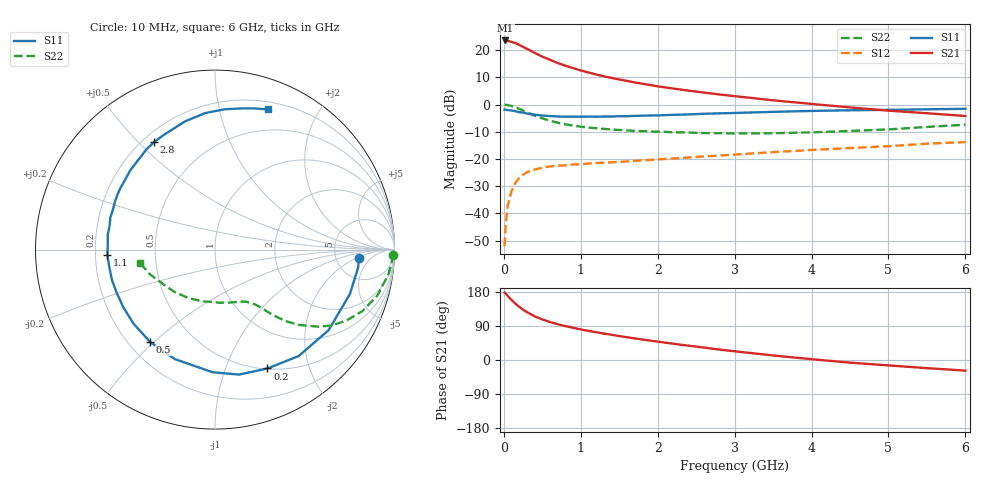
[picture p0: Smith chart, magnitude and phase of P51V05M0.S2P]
! SIEMENS Small Signal Semiconductors
! BFP183
! Si NPN RF Bipolar Junction Transistor in SOT143
! VCE = 1 V  IC = 5 mA
! Common Emitter S-Parameters:  March  1996
# GHz  S  MA  R  50
!  f  S11  S21  S12  S22
! GHz  MAG  ANG  MAG  ANG  MAG  ANG  MAG  ANG
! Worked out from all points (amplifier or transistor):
!   36 points, 10 MHz to 6 GHz, reference 50 ohm
!   highest |S21| = 23.5 dB at 20 MHz (marker M1)
!   |S21| within 3 dB of that: start of sweep to 297.1 MHz
!   unconditionally stable (mu >= 1): 1.46 GHz to end of sweep
!   at 250 MHz: K = 0.21, MSG = 23.5 dB, |S12| = -25.8 dB
!   at 1.4 GHz: K = 0.98, MSG = 15.5 dB, |S12| = -21.2 dB
!   at 6 GHz: K = 1.02, MAG = 3.9 dB, |S12| = -13.8 dB
!   S11 on the Smith chart (normalised r, x): 10 MHz: 8.53, -2.37; 200 MHz: 0.51, -1.41; 500 MHz: 0.29, -0.48; 1.1 GHz: 0.25, -0.02; 2.8 GHz: 0.24, +0.56; 6 GHz: 0.27, +1.41
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0.01  0.8038 -3.5  14.91 178.1  0.0025 86.8  0.9921 -1.6
0.02  0.8034 -7.3  15.03 176.1  0.0051 84.7  0.9894 -3.3
0.05  0.7914 -18.2  14.86 169.0  0.0137 82.7  0.9762 -8.1
0.1  0.776 -35.3  14.13 158.6  0.0256 71.1  0.9402 -15.8
0.15  0.7544 -51.8  13.43 148.7  0.0364 64.6  0.8895 -22.7
0.2  0.7238 -66.2  12.46 140.3  0.0449 57.9  0.8327 -28.3
0.25  0.7091 -79.1  11.42 132.8  0.0514 52.1  0.7757 -33.0
0.3  0.6837 -91.1  10.59 126.4  0.0572 47.9  0.7185 -36.7
0.4  0.6498 -110.2  8.923 115.4  0.0641 40.8  0.6255 -42.1
0.5  0.6284 -125.2  7.577 107.0  0.0691 36.2  0.5566 -45.5
0.6  0.6137 -137.6  6.634 100.3  0.0729 33.1  0.5038 -47.7
0.7  0.6034 -148.0  5.79 94.5  0.0749 31.1  0.463 -49.4
0.9  0.5985 -163.7  4.667 85.1  0.0792 28.7  0.4096 -51.7
1.1  0.6001 -177.2  3.877 76.7  0.0822 27.2  0.3776 -53.9
1.3  0.603 172.1  3.3 69.8  0.0853 26.9  0.357 -56.3
1.6  0.6107 158.8  2.716 60.0  0.0902 27.5  0.3346 -60.1
2.2  0.6467 136.9  1.968 43.0  0.1021 28.1  0.3097 -71.1
2.8  0.6888 119.4  1.532 27.6  0.1155 27.7  0.2976 -85.0
3.5  0.7338 103.1  1.196 12.0  0.1335 26.4  0.297 -104.1
4.5  0.7839 86.0  0.885 -7.0  0.1586 21.9  0.327 -134.0
5.5  0.8167 74.4  0.692 -21.5  0.1905 16.8  0.3874 -159.1
6  0.8348 69.3  0.615 -28.0  0.2044 12.7  0.4253 -170.2
